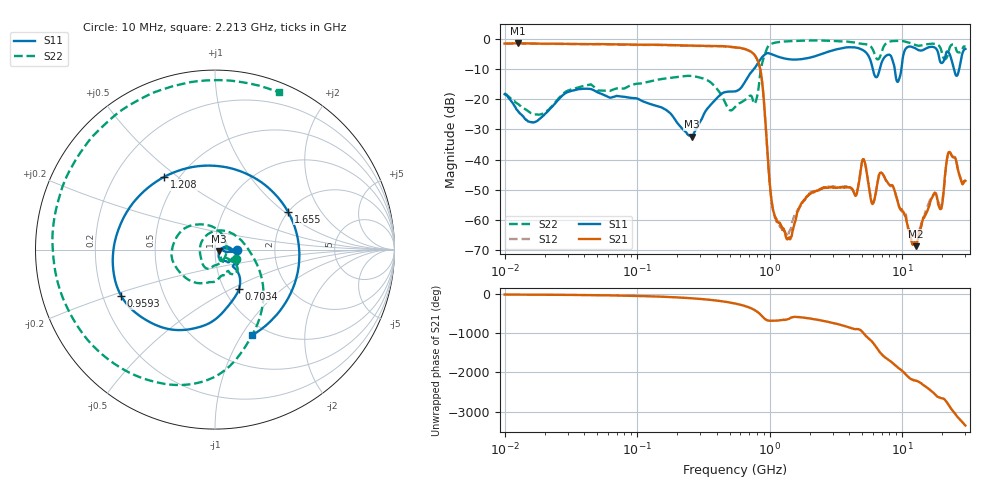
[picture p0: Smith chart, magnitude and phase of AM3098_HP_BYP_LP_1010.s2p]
!Agilent Technologies,E8364B,MY43040894,A.07.50.67
!Agilent E8364B: A.07.50.67
!Date: Wednesday, June 17, 2020 09:21:24
!Correction: S11(Full 2 Port(1,2))
!S21(Full 2 Port(1,2))
!S12(Full 2 Port(1,2))
!S22(Full 2 Port(1,2))
!S2P File: Measurements: S11, S21, S12, S22:Log Frequency Sweep
# Hz S  dB  R 50
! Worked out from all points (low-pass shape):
!   1601 points, 10 MHz to 30 GHz, reference 50 ohm
!   highest |S21| = -1.43 dB at 12.53 MHz (marker M1); lowest = -68.8 dB at 12.69 GHz (marker M2)
!   |S21| within 3 dB of the highest: start of sweep to 734.1 MHz
!   lowest |S11| = -32.4 dB at 257.3 MHz (marker M3), VSWR 1.05, Z = 52.3 - j0.797 ohm
!   |S11| at or under -10 dB: start of sweep to 760.1 MHz; 8.793 GHz to 9.866 GHz (1.073 GHz wide, 11.5 % of centre); 24.62 GHz to 26.93 GHz (2.31 GHz wide, 8.96 % of centre)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
!   |S22| runs from -25.1 to -0.5 dB; largest |S21 - S12| = 0.014
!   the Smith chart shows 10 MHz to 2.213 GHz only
!   S11 on the Smith chart (normalised r, x): 10 MHz: 1.28, -0.01; 703.4 MHz: 1.17, -0.55; 959.3 MHz: 0.28, -0.22; 1.208 GHz: 0.42, +0.45; 1.655 GHz: 1.99, +1.06; 2.213 GHz: 0.85, -1.11
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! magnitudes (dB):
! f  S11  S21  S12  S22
! 10 MHz  -18.3  -1.5  -1.5  -18.0
! 12.53 MHz  -23.7  -1.4  -1.5  -21.5
! 38.04 MHz  -16.6  -1.7  -1.7  -15.8
! 144.7 MHz  -22.4  -1.9  -2.0  -13.5
! 257.3 MHz  -32.4  -2.2  -2.3  -12.3
! 547.7 MHz  -17.4  -2.7  -2.8  -22.6
! 703.4 MHz  -11.8  -3.9  -4.0  -18.9
! 850.8 MHz  -6.8  -10.1  -10.3  -11.2
! 959.3 MHz  -4.7  -36.9  -37.1  -2.9
! 1.055 GHz  -5.2  -56.2  -56.1  -1.4
! 1.208 GHz  -6.1  -61.8  -62.4  -0.9
! 1.655 GHz  -6.8  -56.3  -56.5  -0.6
! 2.084 GHz  -6.0  -50.9  -50.6  -0.5
! 2.213 GHz  -5.7  -50.5  -50.8  -0.5
! 5.103 GHz  -3.8  -39.9  -39.9  -1.7
! 5.959 GHz  -9.4  -54.8  -54.6  -3.2
! 7.926 GHz  -5.2  -48.1  -48.3  -1.0
! 9.302 GHz  -14.2  -54.3  -54.2  -0.7
! 12.69 GHz  -3.2  -68.8  -64.8  -2.0
! 19.7 GHz  -8.0  -56.4  -55.4  -3.7
! 22.56 GHz  -4.6  -37.6  -37.5  -3.7
! 30 GHz  -3.3  -47.0  -47.2  -2.6
